TYPE TMP_IN :
STRUCT
	Rotation	:	BIT	;	//1:ROTATING,0:NOT ROTATING
	Normal	:	BIT	;	//1:NORMAL,0:UNNORMAL
	Acceleration	:	BIT	;	
	Deceleration_Includes_Braking	:	BIT	;	
	Remote_Local	:	BIT	;	//1:LOCAL.E-CAT CONTROL DISABLED,0:REMOTE.E-CAT CONTROL ENABLED
	Turbo_Low_Speed	:	BIT	;	
	Alarm	:	BIT	;	
	Warning	:	BIT	;	
	Turbo_Speed	:	INT	;	//0.1[%],1000(100.0%):RATED SPEED,0(0.0%):NO RATATION
	Turbo_Current	:	INT	;	//0.1A
	Turbo_pump_temperature	:	INT	;	//1[℃]
	VibrationH	:	INT	;	
	VibrationB	:	INT	;	
	VibrationZ	:	INT	;	
END_STRUCT
END_TYPE
